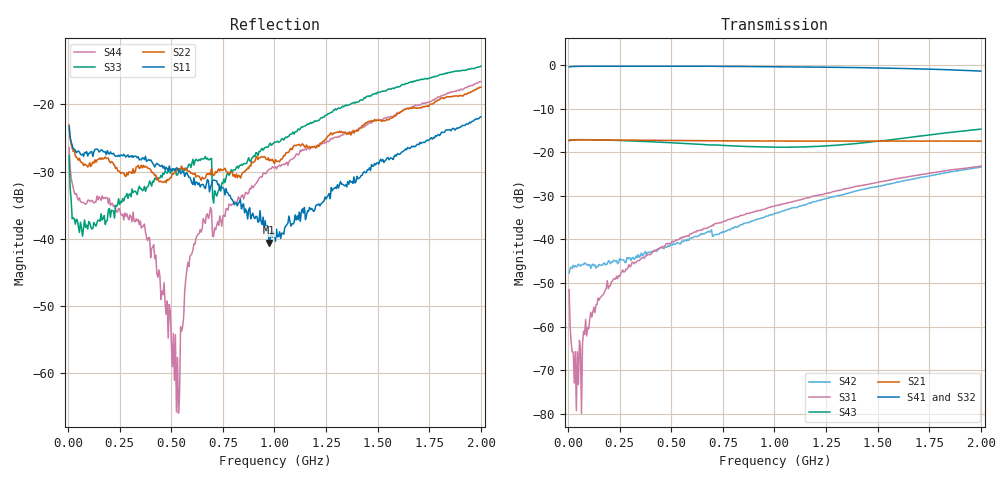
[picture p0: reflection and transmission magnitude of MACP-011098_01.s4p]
!Agilent Technologies,E5071C,MY46110647,A.11.31
!Date: Wed Jul 20 13:22:57 2022
!Data & Calibration Information:
!MACP-011098 solderedd onto PT-0003645 with F connectors, Port1 (pin3) Port2 (pin1) Port3 (pin6) Port4 (pin4)
!Freq	S11:SOLT4(ON)	S12:SOLT4(ON)	S13:SOLT4(ON)	S14:SOLT4(ON)
!	S21:SOLT4(ON)	S22:SOLT4(ON)	S23:SOLT4(ON)	S24:SOLT4(ON)
!	S31:SOLT4(ON)	S32:SOLT4(ON)	S33:SOLT4(ON)	S34:SOLT4(ON)
!	S41:SOLT4(ON)	S42:SOLT4(ON)	S43:SOLT4(ON)	S44:SOLT4(ON)
!PortZ  Port1:75+j0  Port2:75+j0  Port3:75+j0  Port4:75+j0
!Above PortZ is port z conversion or system Z0 setting when saving the data.
!When reading, reference impedance value at option line is always used.
# Hz S MA R 75
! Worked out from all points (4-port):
!   400 points, 5 MHz to 2 GHz, reference 75 ohm
!   strongest paths, dB at 5 MHz, 505 MHz, 1.005 GHz, 1.505 GHz, 2 GHz:
!     S41: -0.5, -0.3, -0.4, -0.7, -1.4
!     S32: -0.5, -0.3, -0.5, -0.7, -1.4
!     S21: -17.4, -17.3, -17.5, -17.5, -17.5
!     S43: -17.3, -17.9, -18.9, -17.5, -14.7
!     S31: -51.5, -40.4, -32.3, -26.9, -23.2
!     S42: -47.7, -41.3, -34.0, -27.8, -23.4
!   lowest |S11| = -40.6 dB at 975 MHz (marker M1), VSWR 1.02, Z = 73.9 - j0.885 ohm
!   |S11| at or under -10 dB: start of sweep to end of sweep
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5000000  0.06855 148.7  0.1344 -176.9  0.004242 -157.9  0.9504 1.9
         0.135 -177.6  0.07005 148.1  0.9465 2.2  0.001754 -74.9
         0.002646 -21.3  0.9487 2.0  0.0416 93.2  0.1398 1.0
         0.9479 2.1  0.004111 -153.8  0.1367 1.4  0.04789 136.4
6.5e7  0.04208 179.8  0.1378 175.5  0.004661 172.9  0.9642 -1.5
       0.1379 175.5  0.03691 175.4  0.964 -1.6  0.001084 128.9
       0.0001016 46.8  0.9637 -1.6  0.01196 33.4  0.1388 -1.0
       0.9637 -1.4  0.005072 176.4  0.1389 -1.1  0.01869 178.0
8.5e7  0.04347 179.6  0.1379 174.0  0.004427 172.0  0.9652 -2.1
       0.1382 173.9  0.0355 173.0  0.9642 -2.3  0.00138 135.8
       0.001209 95.4  0.9643 -2.3  0.01217 40.4  0.1391 -1.5
       0.9644 -2.1  0.005258 170.2  0.1386 -1.6  0.01805 172.6
5.35e8  0.03149 -164.6  0.136 140.9  0.009538 113.8  0.9656 -15.9
        0.1362 140.9  0.03264 -160.3  0.9625 -16.6  0.007333 104.0
        0.009935 80.7  0.9625 -16.6  0.03109 33.7  0.1269 -8.3
        0.9655 -15.9  0.009106 141.3  0.1269 -8.4  0.0005014 132.4
6.2e8  0.02639 -155.9  0.1357 134.9  0.01129 109.4  0.9639 -18.4
       0.1355 135.0  0.02884 -142.9  0.9608 -19.2  0.009816 99.3
       0.01211 78.6  0.9603 -19.3  0.03902 23.6  0.1236 -8.6
       0.9656 -18.4  0.01083 132.6  0.1237 -8.7  0.01018 -20.6
9.75e8  0.009321 -140.0  0.1344 110.5  0.02319 64.7  0.9542 -29.3
        0.1345 110.5  0.03805 -148.1  0.9516 -30.5  0.02007 80.9
        0.02329 64.4  0.9515 -30.5  0.0505 -65.2  0.1141 -5.4
        0.954 -29.3  0.01909 80.0  0.1144 -5.4  0.0329 -51.2
2e9  0.08085 -149.1  0.1345 29.8  0.06814 -13.0  0.85 -63.5
     0.1335 29.3  0.1342 175.3  0.8517 -65.4  0.0666 6.9
     0.06893 -13.0  0.8526 -65.5  0.1925 -120.3  0.1827 -5.7
     0.8495 -63.5  0.06733 7.1  0.1834 -6.1  0.1476 -133.2
